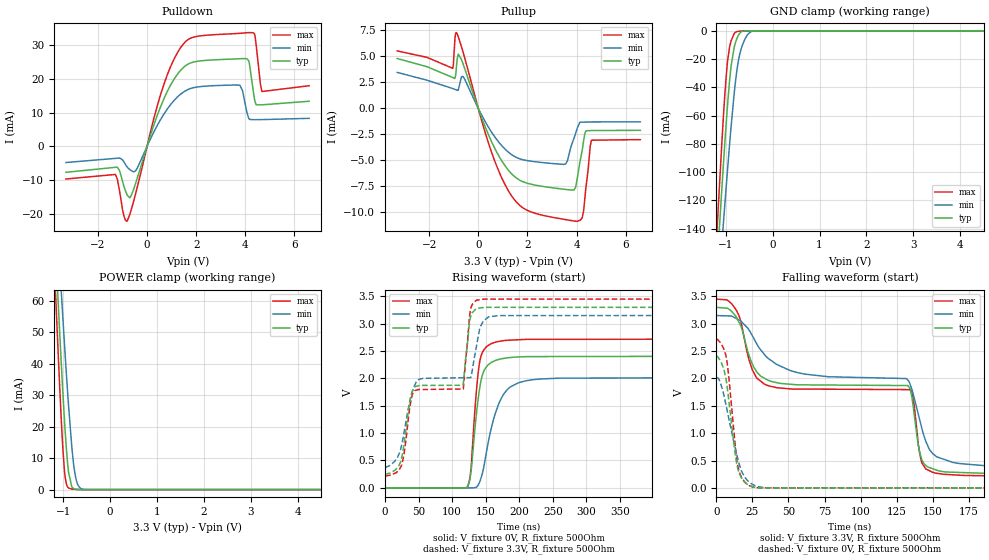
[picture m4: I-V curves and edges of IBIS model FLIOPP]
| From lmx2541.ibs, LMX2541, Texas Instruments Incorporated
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|   Model FLIOPP
[Model]   FLIOPP
Model_type   3-state
Polarity   Non-Inverting
Vmeas = 1.65
Vref = 3.3
Cref = 1pF
Rref = 500
|   typ   min   max
|   (nom PVT)   (fast PVT)   (slow PVT)
C_comp   0.428p   0.419p   0.442p
|C_comp (ON state)   0.425p   0.413p   0.441p
|C_comp (OFF state)   0.428p   0.419p   0.442p
[Voltage Range]   3.3   3.15   3.45
[Temperature Range]   27   125   -40
[Pullup Reference]   3.3   3.15   3.45
[Pulldown Reference]   0   0   0
[Power Clamp Reference]   3.3   3.15   3.45
[GND Clamp Reference]   0   0   0
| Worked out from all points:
|   slope of the pulldown table from 0 to 0.495 V, typ, clamps not added: 46.3 ohm
|   slope of the pullup table from 0 to 0.495 V, typ, clamps not added: 167 ohm
|   GND clamp passes 1 mA (typ) near -0.68 V on its own axis
|   POWER clamp passes 1 mA (typ) near -0.82 V on its own axis
|   falling waveform, V_fixture 3.3V, R_fixture 500Ohm: 20-80 % time 120ns typ, 115ns min, 121ns max; typ from 3.3 V to 0.246 V
|   rising waveform, V_fixture 0V, R_fixture 500Ohm: 20-80 % time 12.8ns typ, 24.8ns min, 10.3ns max; typ from 0 V to 2.4 V
|   rising waveform, V_fixture 3.3V, R_fixture 500Ohm: 20-80 % time 94.2ns typ, 109ns min, 92.7ns max; typ from 0.246 V to 3.3 V
|   falling waveform, V_fixture 0V, R_fixture 500Ohm: 20-80 % time 6.78ns typ, 10.3ns min, 6.07ns max; typ from 2.4 V to 0 V
[Pulldown]
|   Voltage   I(typ)   I(min)   I(max)
-3.3V     -7.679mA   -4.774mA   -9.657mA
-1.293V   -6.194mA   -3.552mA   -8.311mA
-807.7mV  -14.42mA   -6.13mA    -22.12mA
-451.3mV  -10.61mA   -7.078mA   -13.61mA
736.7mV   14.92mA    10.13mA    19.44mA
1.816V    24.84mA    17.26mA    32.19mA
3.776V    25.97mA    18.09mA    33.5mA
4.063V    25.97mA    10.18mA    33.68mA
4.33V     16.1mA     7.922mA    33.67mA
4.449V    12.29mA    7.926mA    29.63mA
4.677V    12.32mA    7.938mA    16.26mA
6.598V    13.37mA    8.316mA    17.98mA
[GND Clamp]
|   Voltage   I(typ)   I(min)   I(max)
-3.3V     -1.383A    -1.212A    -1.541A
-1.184V   -165.8mA   -196.6mA   -140.6mA
-1.164V   -155.1mA   -187.6mA   -128.4mA
-1.085V   -113.1mA   -152mA     -80.86mA
-1.045V   -92.77mA   -134.5mA   -58.76mA
-966.1mV  -54.82mA   -100.5mA   -23.33mA
-886.9mV  -25.31mA   -68.43mA   -7.255mA
-778mV    -6.955mA   -32.12mA   -785uA
-718.6mV  -2.526mA   -19.33mA   -330.1uA
-639.4mV  -313.3uA   -9.741mA   -94.29uA
-401.8mV  -461.1nA   -145.3uA   -134.8nA
6.598V    0A         0A         0A
[Pullup]
|   Voltage   I(typ)   I(min)   I(max)
-3.3V     4.804mA    3.466mA    5.535mA
-1.045V   2.982mA    1.914mA    3.866mA
-886.9mV  4.081mA    1.776mA    7.3mA
-619.6mV  4.284mA    3.08mA     5.419mA
845.6mV   -4.61mA    -3.28mA    -6.099mA
2.152V    -7.294mA   -5.08mA    -9.962mA
3.558V    -7.797mA   -5.333mA   -10.7mA
3.964V    -7.592mA   -2.385mA   -10.86mA
4.132V    -5.208mA   -1.352mA   -10.77mA
4.281V    -3.238mA   -1.316mA   -9.962mA
4.608V    -2.129mA   -1.302mA   -3.059mA
6.598V    -2.108mA   -1.288mA   -3mA
[POWER Clamp]
|   Voltage   I(typ)   I(min)   I(max)
-3.3V     787.6mA    691.1mA    878.1mA
-1.164V   76.78mA    94.56mA    62.67mA
-1.154V   73.73mA    91.97mA    59.2mA
-1.075V   49.88mA    71.51mA    32.58mA
-1.035V   38.51mA    61.52mA    20.57mA
-966.1mV  20.36mA    44.61mA    4.96mA
-886.9mV  5.513mA    26.79mA    507.5uA
-807.7mV  734uA      12.17mA    150.8uA
-748.3mV  159.3uA    4.962mA    78.71uA
-688.9mV  45.34uA    1.579mA    33.67uA
-589.9mV  6.415uA    160.7uA    3.88uA
6.598V    0A         0A         0A
[Ramp]
R_load = 500
|   typ   min   max
dV/dt_r   1.44299/1.27358e-08   1.20738/2.4601e-08   1.63112/1.02858e-08
dV/dt_f   1.83254/1.1969e-07   1.66888/1.1539e-07   1.94202/1.20845e-07
[Falling Waveform]
V_fixture = 3.3V
V_fixture_min = 3.15V
V_fixture_max = 3.45V
R_fixture = 500Ohm
C_fixture = 0F
|   Time   V(typ)   V(min)   V(max)
0s        3.3V       3.15V      3.45V
13.94ns   3.12V      3.095V     3.245V
25.03ns   2.262V     2.777V     2.152V
33.13ns   2.007V     2.445V     1.899V
61.2ns    1.882V     2.079V     1.806V
132.8ns   1.87V      1.969V     1.796V
136ns     1.566V     1.753V     1.703V
142.2ns   526.4mV    1.111V     477.8mV
149.9ns   350.5mV    628.2mV    283.8mV
499.9ns   245.8mV    368.5mV    213.3mV
[Rising Waveform]
V_fixture = 0V
V_fixture_min = 0V
V_fixture_max = 0V
R_fixture = 500Ohm
C_fixture = 0F
|   Time   V(typ)   V(min)   V(max)
0s        1.06uV     1.107nV    280.9pV
122.7ns   23.59mV    -414.8uV   13.84mV
127.9ns   285.8mV    -432.5uV   346mV
135.3ns   1.26V      5.984mV    1.664V
140.5ns   1.792V     96.68mV    2.273V
147ns     2.131V     380.3mV    2.52V
157.4ns   2.284V     1.049V     2.631V
176ns     2.365V     1.703V     2.69V
209.1ns   2.398V     1.955V     2.714V
499.9ns   2.405V     2.012V     2.719V
[Rising Waveform]
V_fixture = 3.3V
V_fixture_min = 3.15V
V_fixture_max = 3.45V
R_fixture = 500Ohm
C_fixture = 0F
|   Time   V(typ)   V(min)   V(max)
0s        245.7mV    368.5mV    213.3mV
25.03ns   569.4mV    802.5mV    423.1mV
37.45ns   1.615V     1.614V     1.519V
43.88ns   1.841V     1.869V     1.777V
116.3ns   1.894V     2.013V     1.808V
127.1ns   3.118V     2.015V     3.257V
136ns     3.277V     2.584V     3.43V
141.9ns   3.29V      2.945V     3.441V
155.3ns   3.3V       3.129V     3.45V
499.9ns   3.3V       3.15V      3.45V
[Falling Waveform]
|Gnd
V_fixture = 0V
V_fixture_min = 0V
V_fixture_max = 0V
R_fixture = 500Ohm
C_fixture = 0F
|   Time   V(typ)   V(min)   V(max)
0s        2.405V     2.012V     2.719V
2.348ns   2.342V     1.95V      2.669V
5.382ns   2.154V     1.679V     2.522V
7.49ns    1.848V     1.414V     2.29V
13.1ns    620mV      728.4mV    780.6mV
15.27ns   316.4mV    494.2mV    353.6mV
19.76ns   102.9mV    193.8mV    104.9mV
25.03ns   21.86mV    64.56mV    17.09mV
43.69ns   80.72uV    116.4uV    69.34uV
499.9ns   1.06uV     38.13nV    120.5nV
